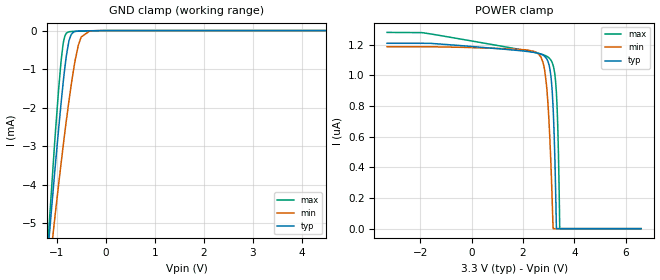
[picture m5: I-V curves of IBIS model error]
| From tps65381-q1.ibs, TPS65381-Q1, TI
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|   error Model
[Model]   error
Model_type   Input
Vinl = 0.99
Vinh = 2.31
|   typ   min   max
|   (nom PVT)   (fast PVT)   (slow PVT)
C_comp   3.865e-13   3.215e-13   3.942e-13
[Model spec]
|subparameter
Vinl   0.99   0.951   1.029
Vinh   2.31   2.219   2.401
| Where nom  PVT is Nominal Process, 3.3V, 27C
|   Fast PVT is Strong Process,  3.43V, -40C
|   Slow PVT is Weak Process,   3.17V, 150C
[Voltage Range]   3.3   3.17   3.43
|Junction Temperature
[Temperature Range]   27   150   -40
[Power Clamp Reference]   3.3   3.17   3.43
[GND Clamp Reference]   0   0   0
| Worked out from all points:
|   GND clamp passes 1 mA (typ) near -0.84 V on its own axis
[GND Clamp]
|   Voltage   I(typ)   I(min)   I(max)
-3.3V     -42.94mA   -34.13mA   -52.97mA
-1.187V   -5.851mA   -6.606mA   -5.669mA
-1.052V   -3.851mA   -5.026mA   -3.113mA
-910.8mV  -1.887mA   -3.449mA   -795.9uA
-871.6mV  -1.395mA   -3.033mA   -369.2uA
-833.8mV  -963.4uA   -2.644mA   -140.5uA
-751.5mV  -273.7uA   -1.84mA    -30.78uA
-703.8mV  -98.92uA   -1.409mA   -23.87uA
-557.9mV  -12.14uA   -378.7uA   -16.72uA
-500.9mV  -9.301uA   -167.7uA   -14.45uA
-330mV    -5.174uA   -13.57uA   -8.195uA
6.6V      0A         0A         0A
[POWER Clamp]
|   Voltage   I(typ)   I(min)   I(max)
-3.3V     1.209uA    1.186uA    1.279uA
2.178V    1.155uA    1.164uA    1.158uA
2.567V    1.144uA    1.144uA    1.144uA
2.835V    1.124uA    1.04uA     1.131uA
2.993V    1.079uA    754.7nA    1.116uA
3.132V    906.9nA    206.9nA    1.084uA
3.173V    782.7nA    0A         1.064uA
3.234V    491.4nA    0A         1.012uA
3.303V    0A         0A         877nA
3.364V    0A         0A         594.6nA
3.43V     0A         0A         0A
6.6V      0A         0A         0A
